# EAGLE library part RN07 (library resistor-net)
RESISTOR NETWORK
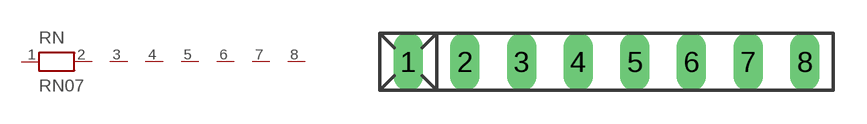
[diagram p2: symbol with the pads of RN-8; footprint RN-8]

Designator prefix RN

## RN07 (OC_FARNELL: unknown; OC_NEWARK: unknown)  [RN-8]
1  1  pas
2  2  pas
3  3  pas
4  4  pas
5  5  pas
6  6  pas
7  7  pas
8  8  pas

## Footprint RN-8 (pad centres in mm)
RESISTOR NETWORK
drill 0.813 long: 1 -8.89,0; 2 -6.35,0; 3 -3.81,0; 4 -1.27,0; 5 1.27,0; 6 3.81,0; 7 6.35,0; 8 8.89,0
